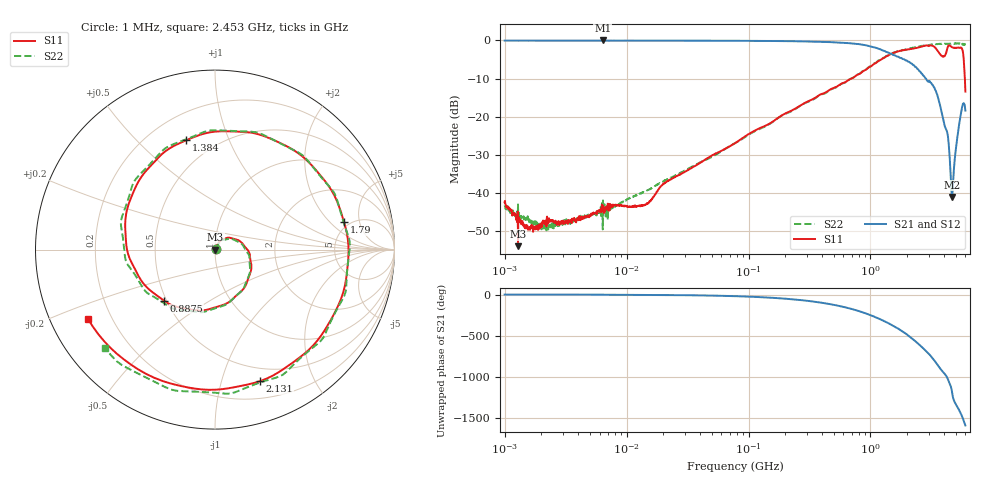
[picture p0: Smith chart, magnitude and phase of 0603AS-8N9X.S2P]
!s-Parameter Generated by FASTRON Sdn. Bhd.
!FASTRON P/N : 0603AS-8N9X
!Keysight Technologies: E5071C_MY46733604_B.14.02
!Date: Mon Dec 04 10:03:00 2023
!Version  :Rev01  Mon Dec 04 10:03:00 2023
!Data & Calibration Information:
!Freq  S11:SOLT2(ON)  S21:SOLT2(ON)  S12:SOLT2(ON)  S22:SOLT2(ON)
!PortZ  Port1:50+j0  Port2:50+j0
!When reading reference impedance value at option line is always used.
! Remarks : This data is being provided solely for informational purposes.
# Hz S dB R 50
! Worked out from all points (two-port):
!   1601 points, 1 MHz to 6 GHz, reference 50 ohm
!   highest |S21| = 0.00 dB at 6.378 MHz (marker M1); lowest = -41.1 dB at 4.657 GHz (marker M2)
!   |S21| within 3 dB of the highest: start of sweep to 1.345 GHz
!   lowest |S11| = -54.0 dB at 1.288 MHz (marker M3), VSWR 1.00, Z = 50.2 + j0.044 ohm
!   |S11| at or under -10 dB: start of sweep to 697.8 MHz; 5.942 GHz to end of sweep
!   |S22| runs from -49.8 to -0.7 dB; largest |S21 - S12| = 0.0092
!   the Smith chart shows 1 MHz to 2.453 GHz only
!   S11 on the Smith chart (normalised r, x): 1 MHz: 1.01, +0.01; 887.5 MHz: 0.48, -0.33; 1.384 GHz: 0.35, +0.71; 1.79 GHz: 4.49, +2.99; 2.131 GHz: 0.36, -1.33; 2.453 GHz: 0.11, -0.25
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1000000  -42.49 23.7  -0.04 -0.1  -0.04 -0.2  -43.28 22.6
1287650  -54.00 12.7  -0.06 -0.2  -0.02 -0.2  -43.02 6.8
4277066  -46.87 46.1  -0.05 -1.1  -0.04 -1.1  -46.70 47.8
6378092  -44.60 60.5  0.00 -1.6  -0.04 -1.8  -49.59 55.5
1.823719e7  -39.14 65.1  -0.05 -4.7  -0.06 -4.7  -37.66 61.2
7.757876e7  -26.95 62.0  -0.09 -19.7  -0.09 -19.7  -26.99 58.5
3.307917e8  -15.53 5.5  -0.28 -82.7  -0.28 -82.7  -15.71 3.2
6.317636e8  -10.82 -68.0  -0.64 -157.6  -0.64 -157.6  -10.87 -67.1
8.87456e8  -7.91 -135.0  -1.18 138.5  -1.18 138.4  -7.84 -127.5
1.383968e9  -4.01 104.8  -3.11 17.6  -3.11 17.6  -3.99 109.4
1.414819e9  -3.83 98.3  -3.26 9.9  -3.26 9.9  -3.84 100.4
1.790488e9  -2.67 12.0  -4.62 -77.1  -4.63 -77.1  -2.72 13.2
2.130642e9  -2.22 -71.1  -5.95 -157.2  -5.95 -157.1  -2.01 -63.0
2.45304e9  -1.87 -151.2  -7.54 126.3  -7.51 126.5  -1.69 -138.2
3.024401e9  -1.41 82.3  -10.67 -0.2  -10.62 -0.4  -1.25 89.7
3.442219e9  -2.09 -22.9  -13.31 -105.7  -13.29 -106.0  -1.00 -6.8
3.847204e9  -4.04 -132.4  -19.19 158.3  -19.22 157.9  -0.94 -101.5
4.211689e9  -2.69 161.2  -23.64 86.4  -23.68 86.1  -0.93 174.2
4.656967e9  -1.76 74.6  -41.06 -98.6  -41.13 -98.7  -0.86 74.5
5.020705e9  -1.92 15.6  -28.30 108.1  -28.34 108.1  -0.82 -2.9
5.384443e9  -1.92 -56.5  -21.23 27.4  -21.27 27.4  -0.77 -81.3
6e9  -13.43 72.6  -18.41 -145.6  -18.44 -145.6  -1.09 153.4
